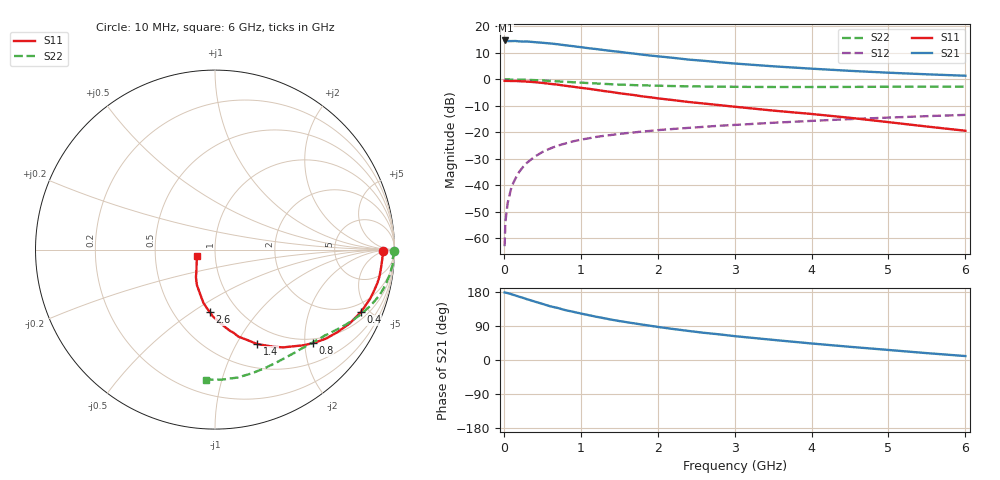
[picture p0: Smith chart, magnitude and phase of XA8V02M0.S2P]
! SIEMENS Discrete & RF Semiconductors
! BFY180
! Si NPN RF Bipolar Junction Transistor in MICRO-X
! VCE = 8 V  IC = 2 mA
! Common Emitter S-Parameters:  May  1997
# GHz  S  MA  R  50
!  f  S11  S21  S12  S22
! GHz  MAG  ANG  MAG  ANG  MAG  ANG  MAG  ANG
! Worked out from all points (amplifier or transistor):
!   36 points, 10 MHz to 6 GHz, reference 50 ohm
!   highest |S21| = 14.7 dB at 20 MHz (marker M1)
!   |S21| within 3 dB of that: start of sweep to 1.124 GHz
!   unconditionally stable (mu >= 1): 3.193 GHz to end of sweep
!   at 250 MHz: K = 0.11, MSG = 23.7 dB, |S12| = -33.1 dB
!   at 1.4 GHz: K = 0.63, MSG = 15.9 dB, |S12| = -21.0 dB
!   at 6 GHz: K = 1.05, MAG = 6.0 dB, |S12| = -13.4 dB
!   S11 on the Smith chart (normalised r, x): 10 MHz: 30, -4; 400 MHz: 1.40, -4.45; 800 MHz: 0.90, -2.18; 1.4 GHz: 0.77, -1.22; 2.6 GHz: 0.74, -0.59; 6 GHz: 0.82, -0.06
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0.01  0.9359 -0.5  5.343 178.2  0.0007 95.1  0.9966 -0.3
0.02  0.9342 -1.1  5.435 177.7  0.002 91.8  0.9963 -0.6
0.05  0.9339 -2.9  5.288 176.6  0.0046 88.6  0.9952 -1.6
0.1  0.9307 -6.1  5.288 173.5  0.0093 86.7  0.9909 -3.3
0.15  0.9289 -9.2  5.308 170.3  0.0132 85.0  0.9931 -4.9
0.3  0.906 -17.8  5.2 160.5  0.0264 78.7  0.9779 -9.5
0.4  0.8841 -23.2  5.048 154.3  0.0344 75.1  0.9661 -12.5
0.6  0.8223 -34.0  4.78 141.9  0.0491 68.8  0.9343 -17.9
0.7  0.7931 -38.7  4.602 137.3  0.0556 65.5  0.9165 -20.4
0.8  0.7547 -43.7  4.409 131.6  0.0613 63.4  0.8977 -22.7
1  0.6917 -51.2  4.059 122.7  0.0723 58.4  0.8656 -26.8
1.1  0.6643 -55.1  3.883 118.5  0.0765 56.4  0.8501 -28.6
1.2  0.6324 -58.9  3.74 114.2  0.0814 54.6  0.8355 -30.4
1.4  0.576 -66.0  3.437 106.4  0.0888 51.6  0.8082 -33.7
1.8  0.4757 -77.3  2.93 93.4  0.103 46.8  0.7703 -39.4
2.2  0.4048 -86.5  2.551 81.9  0.1152 43.0  0.7464 -44.7
2.6  0.349 -94.8  2.241 71.8  0.1264 39.9  0.7304 -49.7
3  0.3034 -102.3  1.991 63.0  0.1373 37.0  0.7218 -54.5
3.5  0.2564 -109.4  1.765 53.1  0.1508 33.6  0.7164 -60.6
4.5  0.1873 -124.6  1.447 34.8  0.177 26.4  0.7192 -73.3
5.5  0.128 -143.2  1.245 18.1  0.2013 18.7  0.7256 -87.0
6  0.1066 -159.7  1.169 10.4  0.2127 14.4  0.7257 -93.9
